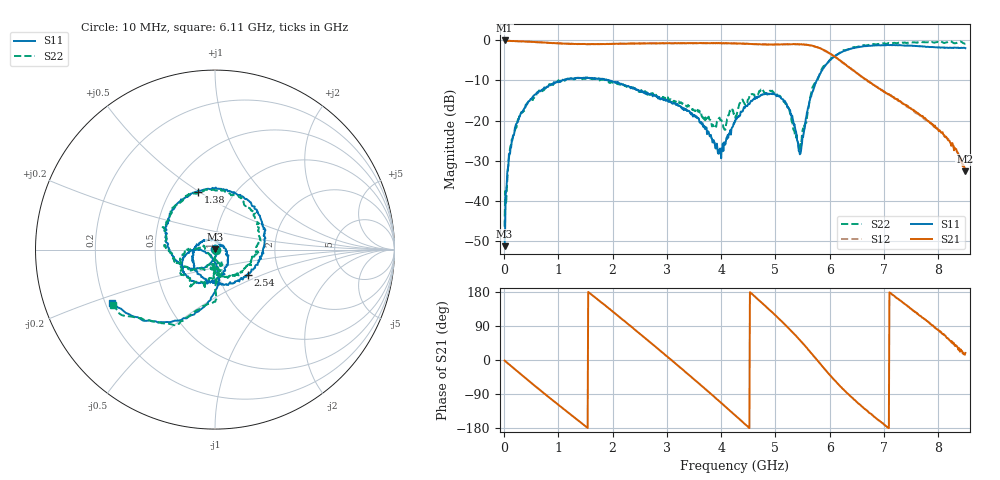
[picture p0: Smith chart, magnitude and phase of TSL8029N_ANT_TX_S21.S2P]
!Agilent Technologies,E5071C,MY46523237,B.13.01
!Date: Wed Aug 16 13:58:42 2023
!Data & Calibration Information:
!Freq	S11:SOLT2(ON)	S21:SOLT2(ON)	S12:SOLT2(ON)	S22:SOLT2(ON)
!PortZ  Port1:50+j0  Port2:50+j0
!Above PortZ is port z conversion or system Z0 setting when saving the data.
!When reading, reference impedance value at option line is always used.
# Hz S dB R 50
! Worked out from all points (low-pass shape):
!   850 points, 10 MHz to 8.5 GHz, reference 50 ohm
!   highest |S21| = -0.06 dB at 10 MHz (marker M1); lowest = -32.6 dB at 8.49 GHz (marker M2)
!   |S21| within 3 dB of the highest: start of sweep to 5.976 GHz
!   lowest |S11| = -51.3 dB at 10 MHz (marker M3), VSWR 1.01, Z = 49.8 + j0.206 ohm
!   |S11| at or under -10 dB: start of sweep to 1.073 GHz; 1.925 GHz to 1.939 GHz (14.45 MHz wide, 0.748 % of centre); 1.941 GHz to 5.761 GHz (3.82 GHz wide, 99.2 % of centre)
!   |S22| runs from -46.4 to -0.2 dB; largest |S21 - S12| = 0.014
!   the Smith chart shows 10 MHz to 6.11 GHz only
!   S11 on the Smith chart (normalised r, x): 10 MHz: 1.00, +0.00; 1.38 GHz: 0.68, +0.50; 2.54 GHz: 1.38, -0.41; 6.11 GHz: 0.23, -0.23
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1e7  -51.26 130.9  -0.06 -1.6  -0.07 -1.5  -46.44 -31.5
1e8  -28.14 -89.7  -0.15 -12.3  -0.16 -12.4  -28.17 -89.0
3.1e8  -18.19 -123.2  -0.28 -37.8  -0.29 -37.6  -18.19 -118.2
8e8  -11.51 175.1  -0.60 -95.2  -0.62 -95.3  -11.50 178.1
1.38e9  -9.47 106.3  -0.92 -161.1  -0.94 -161.3  -9.36 115.1
1.43e9  -9.40 101.1  -0.92 -166.7  -0.92 -166.9  -9.56 110.0
2.08e9  -10.44 22.9  -0.91 119.1  -0.88 118.9  -10.86 41.4
2.54e9  -12.74 -37.8  -0.80 64.5  -0.79 64.8  -12.49 -4.2
2.84e9  -14.52 -81.5  -0.76 28.9  -0.75 29.1  -14.17 -32.4
3.66e9  -20.67 154.4  -0.73 -70.4  -0.72 -70.7  -19.28 -92.2
3.98e9  -26.95 50.2  -0.74 -110.8  -0.73 -110.6  -19.81 -85.3
4.26e9  -20.24 -43.4  -0.79 -146.2  -0.80 -146.7  -19.26 -79.5
4.66e9  -14.43 -108.2  -1.00 162.3  -0.98 162.1  -13.95 -117.6
5.11e9  -14.53 -162.1  -1.01 103.0  -1.03 102.5  -14.41 -167.4
5.45e9  -28.40 -132.3  -1.05 52.5  -1.00 52.6  -26.98 -122.9
5.67e9  -13.31 -87.3  -1.32 16.2  -1.39 16.7  -12.34 -88.8
6.11e9  -3.82 -152.6  -4.27 -56.0  -4.29 -56.8  -3.78 -151.3
6.53e9  -1.71 150.2  -8.47 -114.7  -8.46 -114.6  -1.58 153.6
7.09e9  -1.20 80.2  -13.39 -179.8  -13.54 -179.7  -0.69 96.3
7.77e9  -1.66 -8.7  -19.59 106.1  -19.95 104.8  -0.52 34.9
8.49e9  -1.91 -127.0  -32.64 13.8  -32.28 13.5  -0.88 -36.0
8.5e9  -1.97 -129.0  -32.26 18.7  -32.56 11.4  -0.87 -37.7
